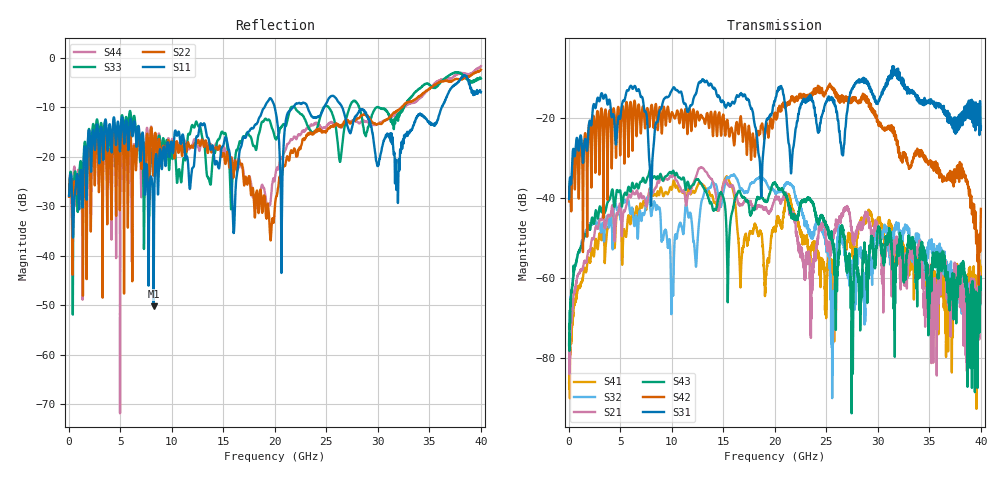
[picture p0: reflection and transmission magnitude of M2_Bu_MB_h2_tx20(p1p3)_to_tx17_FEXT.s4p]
! S11 = S11
! S12 = S12
! S13 = S13
! S14 = S14
! S21 = S21
! S22 = S22
! S23 = S23
! S24 = S24
! S31 = S31
! S32 = S32
! S33 = S33
! S34 = S34
! S41 = S41
! S42 = S42
! S43 = S43
! S44 = S44
! FILE: \\englab.brocade.com\shares\Groups\SIT\Work\Shaohua\IEEE_channels\M2_Bu_MB_h2_tx20(p1p3)_to_tx17_FEXT.s4p
!$DUT_CFG_DESC: Default 4-Port Configuration
!$NUMBER_PORTS: 4
!$DIFF_PORT_MAP: 1|2P|2|2P|0|UC|0|UC|
!$PORT_MAP: PNA 1|1|<<<<<<|TS 2|2|>>>>>>|PNA 2|3|<<<<<<|TS 4|4|>>>>>>|
# MHz S RI R 50.00
! FREQ  S11  S12  S13  S14
!  S21  S22  S23  S24
!  S31  S32  S33  S34
!  S41  S42  S43  S44
!  REAL  IMAG  REAL  IMAG  REAL  IMAG  REAL  IMAG
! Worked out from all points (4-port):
!   3996 points, 50 MHz to 40 GHz, reference 50 ohm
!   strongest paths, dB at 50 MHz, 10.04 GHz, 20.03 GHz, 30.02 GHz, 40 GHz:
!     S31: -40.3, -13.0, -15.7, -16.2, -22.2
!     S42: -40.9, -18.6, -18.8, -21.0, -42.7
!     S43: -76.8, -33.7, -36.4, -48.1, -60.1
!     S21: -72.3, -34.8, -40.2, -48.5, -64.2
!     S32: -76.9, -61.1, -38.7, -49.7, -62.7
!     S41: -86.1, -37.7, -48.2, -45.3, -57.4
!   lowest |S11| = -50.2 dB at 8.25 GHz (marker M1), VSWR 1.01, Z = 50 - j0.306 ohm
!   |S11| at or under -10 dB: start of sweep to 19 GHz; 20 GHz to 21.78 GHz (1.785 GHz wide, 8.55 % of centre); 26.54 GHz to 36.19 GHz (9.652 GHz wide, 30.8 % of centre)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
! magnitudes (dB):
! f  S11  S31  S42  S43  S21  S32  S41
! 50 MHz  -27.9  -40.3  -40.9  -76.8  -72.3  -76.9  -86.1
! 3.22 GHz  -14.6  -13.8  -17.9  -43.6  -45.4  -47.4  -50.3
! 8.25 GHz  -50.2  -27.1  -22.5  -34.7  -38.4  -41.1  -39.4
! 10.05 GHz  -18.2  -13.0  -18.6  -33.6  -34.7  -60.5  -37.6
! 19.67 GHz  -8.3  -19.1  -20.5  -37.6  -42.9  -37.5  -49.6
! 28.67 GHz  -10.8  -11.2  -14.4  -52.7  -44.7  -64.6  -46.1
! 40 GHz  -6.9  -22.2  -42.7  -60.1  -64.2  -62.7  -57.4
